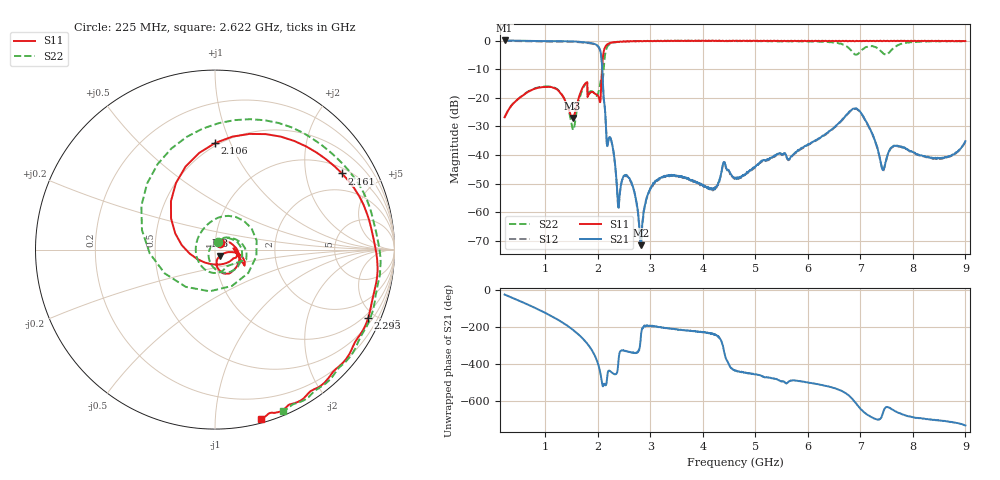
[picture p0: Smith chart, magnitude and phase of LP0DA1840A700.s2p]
!Agilent Technologies,E8358A,US41080443,A.07.50.56
!Agilent E8358A: A.07.50.56
!Date: Wednesday, August 24, 2016 14:48:41
!Correction: S11(Full 2 Port(1,2))
!S21(Full 2 Port(1,2))
!S12(Full 2 Port(1,2))
!S22(Full 2 Port(1,2))
!S2P File: Measurements: S11, S21, S12, S22:
# Hz S  dB  R 50
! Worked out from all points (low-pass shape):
!   1601 points, 225 MHz to 9 GHz, reference 50 ohm
!   highest |S21| = 0.03 dB at 225 MHz (marker M1); lowest = -71.5 dB at 2.819 GHz (marker M2)
!   |S21| within 3 dB of the highest: start of sweep to 2.037 GHz
!   lowest |S11| = -27.0 dB at 1.519 GHz (marker M3), VSWR 1.09, Z = 52.8 - j3.62 ohm
!   |S11| at or under -10 dB: start of sweep to 2.08 GHz
!   |S22| runs from -31.2 to 0.0 dB; largest |S21 - S12| = 0.019
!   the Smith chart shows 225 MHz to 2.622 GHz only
!   S11 on the Smith chart (normalised r, x): 225 MHz: 1.05, +0.08; 2.106 GHz: 0.48, +0.88; 2.161 GHz: 1.20, +3.20; 2.293 GHz: 0.77, -4.59; 2.622 GHz: 0.03, -1.31
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2.25e8  -26.80 56.6  0.03 -26.9  -0.12 -26.7  -26.75 69.2
8.83125e8  -16.46 -30.0  -0.17 -109.2  -0.32 -108.9  -16.31 -8.2
1.519312e9  -27.03 -50.2  -0.29 145.2  -0.45 145.4  -30.72 172.3
1.689328e9  -17.33 -10.6  -0.52 103.3  -0.67 103.6  -17.98 27.6
1.936125e9  -18.43 -23.1  -1.18 8.8  -1.33 9.1  -18.68 -134.5
2.106141e9  -4.52 89.8  -18.82 -155.1  -18.96 -155.1  -11.58 -128.1
2.160984e9  -1.67 30.9  -32.14 -148.7  -32.27 -148.5  -3.04 88.2
2.292609e9  -0.59 -23.9  -38.10 -91.0  -38.26 -90.7  -0.75 -0.3
2.396812e9  -0.47 -46.1  -58.46 -8.4  -58.16 -10.2  -0.49 -30.6
2.621672e9  -0.21 -74.9  -49.01 23.3  -49.13 22.4  -0.19 -67.2
2.819109e9  -0.16 -90.8  -71.55 106.3  -69.50 103.8  -0.14 -87.2
3.153656e9  -0.15 -108.7  -48.48 159.3  -48.30 158.3  -0.11 -110.9
4.6125e9  -0.14 -143.3  -48.08 -74.0  -48.24 -75.1  -0.14 175.6
6.076828e9  -0.07 -170.8  -35.55 -143.1  -35.79 -143.2  -0.38 74.9
6.674625e9  -0.13 175.9  -27.19 170.5  -27.37 171.4  -1.41 0.0
6.855609e9  -0.09 173.0  -23.86 129.4  -24.07 129.9  -4.18 -83.1
6.987234e9  -0.09 170.4  -24.63 84.2  -24.83 84.2  -4.08 163.8
7.146281e9  -0.21 166.9  -29.60 45.0  -29.70 45.5  -2.08 84.2
7.343719e9  -0.19 163.8  -38.87 21.2  -38.97 21.4  -2.81 8.7
7.541156e9  -0.21 160.2  -38.88 86.7  -39.00 86.9  -4.34 -138.2
7.919578e9  -0.13 154.3  -38.35 38.4  -38.50 38.6  -0.71 105.3
9e9  -0.17 137.0  -35.12 -10.1  -35.25 -10.5  -0.22 44.5
